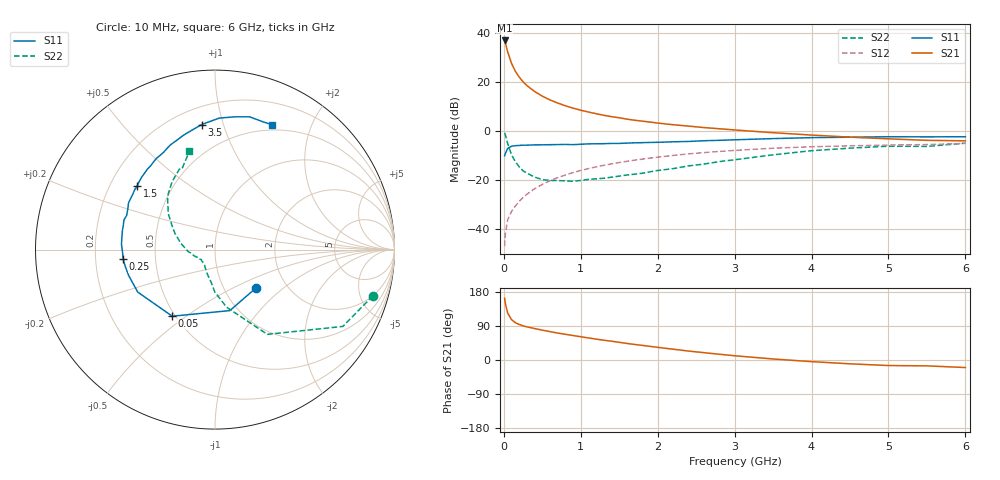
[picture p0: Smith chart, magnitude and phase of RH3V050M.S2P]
! SIEMENS Small Signal Semiconductors
! BFR106
! Si NPN RF Bipolar Junction Transistor in SOT23
! VCE = 3 V  IC = 50 mA
! Common Emitter S-Parameters:  August  1996
# GHz  S  MA  R  50
!  f  S11  S21  S12  S22
! GHz  MAG  ANG  MAG  ANG  MAG  ANG  MAG  ANG
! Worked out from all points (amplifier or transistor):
!   36 points, 10 MHz to 6 GHz, reference 50 ohm
!   highest |S21| = 36.9 dB at 10 MHz (marker M1)
!   |S21| within 3 dB of that: start of sweep to 36.65 MHz
!   unconditionally stable (mu >= 1): 236.2 MHz to 2.461 GHz; 5.481 GHz to 5.602 GHz
!   at 250 MHz: K = 1.01, MAG = 22.9 dB, |S12| = -27.1 dB
!   at 1.4 GHz: K = 1.06, MAG = 8.2 dB, |S12| = -13.4 dB
!   at 6 GHz: K = 1.00, MSG = 0.5 dB, |S12| = -5.0 dB
!   S11 on the Smith chart (normalised r, x): 10 MHz: 1.41, -0.67; 50 MHz: 0.48, -0.44; 250 MHz: 0.32, -0.05; 1.5 GHz: 0.32, +0.32; 3.5 GHz: 0.31, +0.85; 6 GHz: 0.44, +1.46
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0.01  0.313 -42.8  70.11 162.8  0.0045 81.6  0.9166 -16.3
0.02  0.3497 -76.3  62.82 149.0  0.0081 72.3  0.8311 -31.0
0.05  0.441 -122.7  41.09 123.6  0.0155 59.9  0.5549 -58.3
0.1  0.4913 -151.2  23.9 106.5  0.0229 62.0  0.328 -78.5
0.15  0.5023 -163.3  16.47 98.4  0.0296 64.4  0.2371 -90.2
0.2  0.5089 -169.5  12.56 93.8  0.0368 67.1  0.1856 -96.3
0.25  0.5149 -174.2  10.08 90.1  0.0441 68.9  0.1542 -103.7
0.3  0.5146 -177.5  8.443 87.5  0.0515 69.9  0.1385 -108.8
0.4  0.5217 176.9  6.392 83.0  0.0667 71.4  0.115 -118.0
0.5  0.5232 172.8  5.134 78.8  0.0818 71.5  0.1022 -124.9
0.6  0.5267 168.3  4.306 74.9  0.0972 70.8  0.0986 -129.5
0.7  0.5289 164.8  3.721 71.1  0.1121 69.8  0.0976 -135.1
0.8  0.5335 162.1  3.268 67.8  0.1269 68.6  0.0964 -140.5
0.9  0.5277 158.7  2.926 64.6  0.1423 67.7  0.0947 -144.5
1.1  0.5474 151.7  2.438 58.2  0.1713 65.0  0.1034 -150.7
1.5  0.5592 140.9  1.862 46.7  0.2279 59.0  0.1206 -162.9
2.2  0.6032 123.0  1.343 28.5  0.3182 47.8  0.1712 175.6
2.8  0.6461 109.0  1.113 15.2  0.3832 38.2  0.238 158.5
3.5  0.7008 96.1  0.924 2.7  0.446 27.4  0.3275 142.6
4.5  0.7483 81.4  0.75 -10.1  0.4991 13.0  0.4475 122.3
5.5  0.7605 69.7  0.646 -15.5  0.5294 3.8  0.4854 112.3
6  0.7647 65.6  0.631 -19.9  0.5598 -3.2  0.5662 104.6
